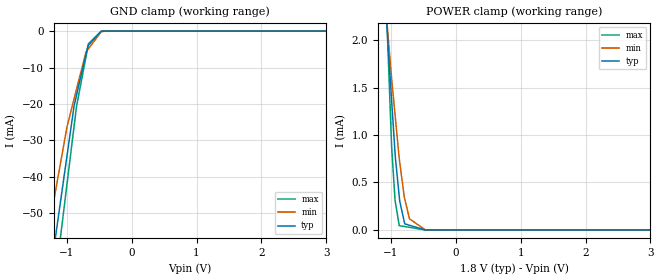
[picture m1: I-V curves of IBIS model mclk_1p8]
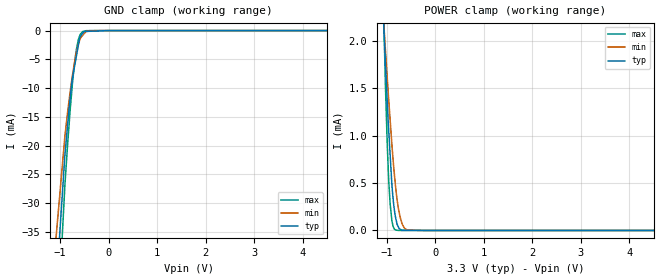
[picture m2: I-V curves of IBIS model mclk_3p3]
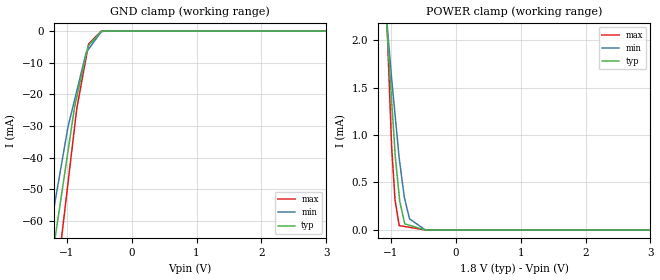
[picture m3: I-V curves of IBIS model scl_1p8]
|Texas Instruments Incorporated
| Low-Power Stereo Codec with 6 Inputs, 6 Outputs, Speaker/HP Amp and
| Enhanced Digital Effects
| Marketing part#   Digital Voltage Range   Package-type   #pins
| TLV320AIC3105IRHBR   1.1V - 3.6V   QFN   32
| TLV320AIC3105IRHBT   1.1V - 3.6V   QFN   32
| TLVAIC3105IRHBRG4   1.1V - 3.6V   QFN   32
| TLVAIC3105IRHBTG4   1.1V - 3.6V   QFN   32
[IBIS Ver]   4.1
[File name]   tlv320aic3105.ibs
[File Rev]   1.1
[Date]   11/15/2012
[Source]
| Texas Instruments Incorporated.
| Analog-eLab Design Center, HPA
| 12500 TI Blvd
| Dallas, TX -75243
| e-mail: elab_scm_ibis@list.ti.com
[Notes]   Revision History:
| Rev 1.1: 10/26/2012
| - Voltage range for modeling is changed for 3.3V models.
| Rev 1.0: 10/23/2012
| - Initial version of the model
| - Model generated from simulations in TISPICE
| - Model matched to SPICE simulation
| - C_comp although listed in numerical order of value are
|   obtained from varying PVT conditions. For PVT conditions for
|   each specific value refer the buffer description under
|   respective [Model]. IBIS model user is responsible for using
|   appropriate C_comp to simulate for Signal Integrity.
| - Model names with a trailing _1p8 contains the model for
|   1.8V [1.71V and 1.89V].Model names with a trailing _3p3
|   contains the model for 3.3V [2.7V and 3.6V].
| - The buffer characteristics for buffer on Pins (MCLK),
|   (DIN) and (_RESET) is same, hence replaced by a single model "mclk".
[Disclaimer]
| This model is designed as an aid for customers of Texas Instruments.
| TI and its licensors and suppliers make no warranties, either expressed
| or implied, with respect to this  model, including the warranties of
| merchantability or fitness for a particular purpose. The model is
| provided solely on an "as is" basis. The entire risk as to its quality
| and performance is with the customer.
[Copyright]
(C) Copyright 2012 Texas Instruments Incorporated.All rights reserved.
|   TLV320AIC3105
[Component]   TLV320AIC3105
[Manufacturer]   TI
[Package]   |32 QFN   -  RHB package
|   typ   min   max
R_pkg   0.0906   0.0381   0.1618
L_pkg   1.3043nH   0.7279nH   2.3304nH
C_pkg   0.1305pF   0.0990pF   0.1822pF
[Pin]  signal_name   model_name   R_pin   L_pin   C_pin
1   MCLK   MCLK   0.08447   1.12717nH   0.10742pF
2   BCLK   BW_CLK   0.07684   1.0114nH   0.11002pF
3   WCLK   BW_CLK   0.07525   0.9891nH   0.10874pF
4   DIN   MCLK   0.081   1.07632nH   0.10073pF
5   DOUT   DOUT   0.09233   1.24893nH   0.12325pF
6   DVSS   GND   0.04303   0.79815nH   0.13999pF
7   IOVDD   POWER   0.09381   1.27233nH   0.12477pF
8   SCL   SCL   0.10744   1.48368nH   0.11004pF
9   SDA   SDA   0.11556   1.61107nH   0.14603pF
10   MIC1LP/LINE1LP   TERM   0.16178   2.33042nH   0.17157pF
11   MIC1LM/LINE1LM   TERM   0.14717   2.10063nH   0.18219pF
12   MIC1RP/LINE1RP   TERM   0.13349   1.88662nH   0.15487pF
13   MIC1RM/LINE1RM   TERM   0.12003   1.67713nH   0.15672pF
14   MIC2L/LINE2L/MICDET   TERM   0.05567   1.1903nH   0.17588pF
15   MICBIAS   TERM   0.10488   1.44363nH   0.12674pF
16   MIC2R/LINE2R   TERM   0.11395   1.58668nH   0.119pF
17   AVSS1   GND   0.11165   1.55027nH   0.14839pF
18   DRVDD   POWER   0.05606   1.27111nH   0.17097pF
19   HPLOUT   TERM   0.09468   1.28503nH   0.13843pF
20   HPLCOM   TERM   0.0802   1.06423nH   0.10312pF
21   DRVSS   GND   0.03807   0.72794nH   0.14057pF
22   HPRCOM   TERM   0.07703   1.01377nH   0.10144pF
23   HPROUT   TERM   0.08826   1.18163nH   0.12835pF
24   DRVDD   POWER   0.05185   1.13694nH   0.14568pF
25   AVDD   POWER   0.09159   1.23347nH   0.12834pF
26   AVSS2   GND   0.0827   1.09612nH   0.09902pF
27   LEFT_LOP   TERM   0.08262   1.09453nH   0.11549pF
28   LEFT_LOM   TERM   0.09107   1.22292nH   0.11081pF
29   RIGHT_LOP   TERM   0.09736   1.31943nH   0.13296pF
30   RIGHT_LOM   TERM   0.11509   1.59373nH   0.13209pF
31   _RESET   MCLK   0.09043   1.21371nH   0.10153pF
32   DVDD   POWER   0.04479   0.89854nH   0.12064pF
|   Model Selectors
[Model Selector] MCLK
mclk_1p8  1.8V digital input
mclk_3p3  3.3V digital input
[Model Selector] SCL
scl_1p8  1.8V digital input
scl_3p3  3.3V digital input
[Model Selector] DOUT
dout_1p8  1.8V digital 3-state
dout_3p3  3.3V digital 3-state
[Model Selector] BW_CLK
bw_clk_1p8  1.8V digital I/O
bw_clk_3p3  3.3V digital I/O
[Model Selector] SDA
sda_1p8  1.8V digital I/O Open Drain
sda_3p3  3.3V digital I/O Open Drain
[Model Selector] TERM
term_1-8V  1.8V nominal termination
term_3-3V  3.3V nominal termination
[Model] term_1-8V
Model_type Terminator
C_comp   1.0e-20F  1.0e-20F  1.0e-20F
|   typ   min   max
[Voltage Range]   1.8V   1.71V   1.89V
[POWER Clamp Reference]   1.8V   1.71V   1.89V
[GND Clamp Reference]   0V   0V   0V
|Ambient Temperature   25   85   -40
|Junction Temperature
[Temperature Range]   27   105   -40
[Model] term_3-3V
Model_type Terminator
C_comp   1.0e-20F  1.0e-20F  1.0e-20F
|   typ   min   max
[Voltage Range]   3.3V   2.7   3.6V
[POWER Clamp Reference]   3.3V   2.7   3.6V
[GND Clamp Reference]   0V   0V   0V
|Ambient Temperature   25   85   -40
|Junction Temperature
[Temperature Range]   27   105   -40
| Models and submodels in the file (12): mclk_1p8 (Input), mclk_3p3 (Input), scl_1p8 (Input), scl_3p3 (Input), dout_1p8 (3-state), dout_3p3 (3-state), bw_clk_1p8 (I/O), bw_clk_3p3 (I/O), sda_1p8 (I/O_open_drain), sda_3p3 (I/O_open_drain), term_1-8V (Terminator), term_3-3V (Terminator)
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|   mclk_1p8 Model
[Model]   mclk_1p8
Model_type   Input
Vinl = 0.54
Vinh = 1.26
|   typ   min   max
|   (nom PVT)   (fast PVT)   (slow PVT)
C_comp   1.043e-12   1.039e-12   1.043e-12
| Where nom  PVT is Nominal Process, 1.8V, 27C
|   Fast PVT is Strong Process,  1.89V, -40C
|   Slow PVT is Weak Process,   1.71V, 105C
[Model Spec]
|Subparameter   typ   min   max
Vinh   1.26   1.197   1.323
Vinl   0.54   0.513   0.567
[Voltage Range]   1.8   1.71   1.89
|Ambient Temperature   25   85   -40
|Junction Temperature
[Temperature Range]   27   105   -40
[Power Clamp Reference]   1.8   1.71   1.89
[GND Clamp Reference]   0   0   0
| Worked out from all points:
|   GND clamp passes 1 mA (typ) near -0.52 V on its own axis
|   POWER clamp passes 1 mA (typ) near -0.96 V on its own axis
[GND Clamp]
|   Voltage   I(typ)   I(min)   I(max)
-1.8V     -243.1mA   -121.9mA   -355.9mA
-1.51V    -98.55mA   -77.34mA   -126.4mA
-1.155V   -54.02mA   -41.99mA   -64.87mA
-996.9mV  -34.24mA   -26.29mA   -41.97mA
-885.6mV  -20.34mA   -18.46mA   -25.83mA
-848.6mV  -17.49mA   -15.86mA   -20.5mA
-704.5mV  -6.404mA   -5.754mA   -7.113mA
-673.2mV  -3.994mA   -5.009mA   -4.203mA
-665.3mV  -3.84mA    -4.821mA   -3.467mA
-470.6mV  -70.83uA   -188.8uA   -24.2uA
-287.3mV  -445.8nA   -2.215uA   -13.16nA
3.6V      0A         0A         0A
[POWER Clamp]
|   Voltage   I(typ)   I(min)   I(max)
-1.8V     11.74mA    8.633mA    19.35mA
-1.081V   2.386mA    2.338mA    2.535mA
-1.04V    1.89mA     2.005mA    1.793mA
-990.4mV  1.367mA    1.596mA    886.6uA
-937.4mV  814.2uA    1.215mA    315.3uA
-930.6mV  748.9uA    1.166mA    286.6uA
-873.2mV  356.4uA    756.1uA    45.76uA
-865.8mV  305.9uA    716.4uA    44.92uA
-788.4mV  64.55uA    328.2uA    36.12uA
-714.8mV  49.55uA    117.7uA    27.76uA
-470.3mV  0A         256.8nA    0A
3.6V      0A         0A         0A
|   mclk_3p3 Model
[Model]   mclk_3p3
Model_type   Input
Vinl = 0.99
Vinh = 2.31
|   typ   min   max
|   (nom PVT)   (fast PVT)   (slow PVT)
C_comp   9.787e-13   9.710e-13   9.903e-13
| Where nom  PVT is Nominal Process, 3.3V, 27C
|   Fast PVT is Strong Process,  3.6V, -40C
|   Slow PVT is Weak Process,   2.7V, 105C
[Model Spec]
|Subparameter   typ   min   max
Vinh   2.31   1.89   2.52
Vinl   0.99   0.81   1.08
[Voltage Range]   3.3   2.7   3.6
|Ambient Temperature   25   85   -40
|Junction Temperature
[Temperature Range]   27   105   -40
[Power Clamp Reference]   3.3   2.7   3.6
[GND Clamp Reference]   0   0   0
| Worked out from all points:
|   GND clamp passes 1 mA (typ) near -0.58 V on its own axis
|   POWER clamp passes 1 mA (typ) near -0.96 V on its own axis
[GND Clamp]
|   Voltage   I(typ)   I(min)   I(max)
-3.3V     -1.786A    -1.575A    -1.965A
-1.498V   -98.66mA   -76.19mA   -123.5mA
-897.6mV  -21.53mA   -18.27mA   -26.74mA
-842.4mV  -16.36mA   -14.17mA   -19.75mA
-772.2mV  -10.33mA   -9.522mA   -12.04mA
-745.8mV  -8.373mA   -7.959mA   -9.433mA
-702mV    -6.326mA   -5.63mA    -5.815mA
-622.8mV  -2.623mA   -2.458mA   -1.616mA
-590.7mV  -1.122mA   -1.587mA   -839.1uA
-532.8mV  -494.1uA   -836.1uA   -172.5uA
-286.2mV  -88.77uA   -2.151uA   -5.093uA
6.6V      0A         0A         0A
[POWER Clamp]
|   Voltage   I(typ)   I(min)   I(max)
-3.3V     32.15mA    22.38mA    56.05mA
-1.076V   2.305mA    2.283mA    2.475mA
-1.03V    1.766mA    1.906mA    1.532mA
-993.6mV  1.375mA    1.621mA    934uA
-964.8mV  1.081mA    1.4mA      561.5uA
-932.4mV  796.9uA    1.166mA    280.4uA
-881.1mV  387.7uA    807.4uA    64.82uA
-820.8mV  138.7uA    461.6uA    4.877uA
-766.8mV  41.34uA    246.3uA    409.3nA
-718.2mV  11.1uA     124.3uA    128.1nA
-583.2mV  2.076uA    6.133uA    0A
6.6V      0A         0A         0A
|   scl_1p8 Model
[Model]   scl_1p8
Model_type   Input
Vinl = 0.54
Vinh = 1.26
|   typ   min   max
|   (nom PVT)   (fast PVT)   (slow PVT)
C_comp   1.183e-12   1.183e-12   1.188e-12
| Where nom  PVT is Nominal Process, 1.8V, 27C
|   Fast PVT is Strong Process,  1.89V, -40C
|   Slow PVT is Weak Process,   1.71V, 105C
[Model Spec]
|Subparameter   typ   min   max
Vinh   1.26   1.197   1.323
Vinl   0.54   0.513   0.567
[Voltage Range]   1.8   1.71   1.89
|Ambient Temperature   25   85   -40
|Junction Temperature
[Temperature Range]   27   105   -40
[Power Clamp Reference]   1.8   1.71   1.89
[GND Clamp Reference]   0   0   0
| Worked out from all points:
|   GND clamp passes 1 mA (typ) near -0.51 V on its own axis
|   POWER clamp passes 1 mA (typ) near -0.96 V on its own axis
[GND Clamp]
|   Voltage   I(typ)   I(min)   I(max)
-1.8V     -260.7mA   -144.7mA   -374.8mA
-1.504V   -119.2mA   -92.4mA    -151.4mA
-1.177V   -65.03mA   -53.51mA   -83.53mA
-1.136V   -59.32mA   -48.6mA    -74.96mA
-983.2mV  -38.24mA   -30.45mA   -48.37mA
-878.4mV  -23.8mA    -21.63mA   -30.1mA
-844.8mV  -20.71mA   -18.82mA   -24.3mA
-701.1mV  -7.468mA   -6.764mA   -8.279mA
-671.4mV  -4.732mA   -5.922mA   -4.969mA
-663.4mV  -4.546mA   -5.695mA   -4.076mA
-470.6mV  -85.43uA   -227.6uA   -29.15uA
3.6V      0A         0A         0A
[POWER Clamp]
|   Voltage   I(typ)   I(min)   I(max)
-1.8V     11.74mA    8.633mA    19.35mA
-1.081V   2.386mA    2.338mA    2.535mA
-1.04V    1.89mA     2.005mA    1.793mA
-990.4mV  1.367mA    1.596mA    886.6uA
-937.4mV  814.2uA    1.215mA    315.3uA
-930.6mV  748.9uA    1.166mA    286.6uA
-873.2mV  356.4uA    756.1uA    45.76uA
-865.8mV  305.9uA    716.4uA    44.92uA
-788.4mV  64.55uA    328.2uA    36.12uA
-714.8mV  49.55uA    117.7uA    27.76uA
-470.3mV  0A         257nA      0A
3.6V      0A         0A         0A
